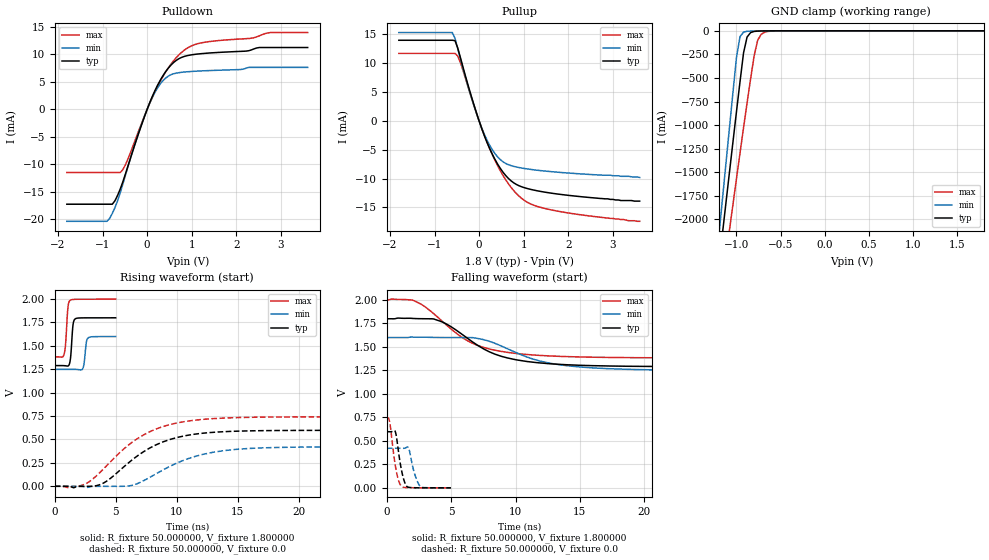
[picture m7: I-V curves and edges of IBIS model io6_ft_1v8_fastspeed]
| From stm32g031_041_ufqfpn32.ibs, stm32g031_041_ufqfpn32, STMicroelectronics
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|   Model io6_ft_1v8_fastspeed
[Model]  io6_ft_1v8_fastspeed
Model_type I/O
Polarity   Non-Inverting
Enable   Active-Low
Vinl =   0.540000V
Vinh =   1.260000V
Vmeas =  0.900000V
Cref =   30.000000pF
Rref =   100.000000M
Vref =   0.0V
C_comp   1.277600pF   1.236700pF   1.315100pF
[Temperature Range]   25.000000   -40.000000   0.125000k
[Pullup Reference]   1.800000V   1.600000V   2.000000V
[Pulldown Reference]   0.0V   0.0V   0.0V
[POWER Clamp Reference]   1.800000V   1.600000V   2.000000V
[GND Clamp Reference]   0.0V   0.0V   0.0V
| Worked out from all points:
|   slope of the pulldown table from 0 to 0.27 V, typ, clamps not added: 54.7 ohm
|   slope of the pullup table from 0 to 0.27 V, typ, clamps not added: 50.6 ohm
|   GND clamp passes 1 mA (typ) near -0.66 V on its own axis
|   rising waveform, R_fixture 50.000000, V_fixture 1.800000: 20-80 % time 165ps typ, 169ps min, 180ps max; typ from 1.29 V to 1.8 V
|   rising waveform, R_fixture 50.000000, V_fixture 0.0: 20-80 % time 4.07ns typ, 4.38ns min, 4.26ns max; typ from 0 V to 0.598 V
|   falling waveform, R_fixture 50.000000, V_fixture 1.800000: 20-80 % time 3.95ns typ, 4.46ns min, 3.82ns max; typ from 1.8 V to 1.29 V
|   falling waveform, R_fixture 50.000000, V_fixture 0.0: 20-80 % time 437ps typ, 479ps min, 450ps max; typ from 0.598 V to 0 V
[Pulldown]
|Voltage   I(typ)   I(min)   I(max)
-1.8V     -17.22mA   -20.33mA   -11.45mA
-900mV    -17.22mA   -20.33mA   -11.45mA
-720mV    -16.58mA   -17.82mA   -11.45mA
-600mV    -14.41mA   -15.08mA   -11.45mA
-480mV    -11.58mA   -11.79mA   -9.954mA
0V        10fA       11fA       0A
240mV     4.49mA     3.999mA    4.291mA
480mV     7.563mA    6.085mA    7.612mA
780mV     9.487mA    6.76mA     10.43mA
1.14V     10.08mA    6.976mA    11.96mA
2.76V     11.26mA    7.652mA    13.98mA
3.6V      11.26mA    7.652mA    13.98mA
[Pullup]
|Voltage   I(typ)   I(min)   I(max)
-1.8V     14mA       15.34mA    11.72mA
-600mV    14mA       15.34mA    11.72mA
-540mV    13.93mA    14.32mA    11.72mA
-420mV    11.01mA    10.78mA    10.15mA
-180mV    4.421mA    4.232mA    4.225mA
60mV      -1.349mA   -1.244mA   -1.314mA
300mV     -5.831mA   -5.038mA   -5.917mA
600mV     -9.499mA   -7.385mA   -10.25mA
960mV     -11.43mA   -8.172mA   -13.47mA
1.32V     -12.13mA   -8.557mA   -14.86mA
2.16V     -13.03mA   -9.116mA   -16.14mA
3.6V      -13.9mA    -9.8mA     -17.4mA
[GND_clamp]
|Voltage   I(typ)   I(min)   I(max)
-1.8V     -7.471A    -7.973A    -7.298A
-1.2V     -2.489A    -2.18A     -2.954A
-1.16V    -2.16A     -1.797A    -2.674A
-1.08V    -1.505A    -1.034A    -2.118A
-1V       -857.9mA   -283.1mA   -1.568A
-960mV    -540.4mA   -62.14mA   -1.296A
-920mV    -234.4mA   -13.75mA   -1.028A
-880mV    -66.29mA   -4.855mA   -765.3mA
-800mV    -6.505mA   -2.056mA   -266mA
-760mV    -3.074mA   -1.45mA    -100.4mA
-680mV    -1.215mA   -557.1uA   -14.19mA
1.8V      0A         0A         0A
[POWER_clamp]
|Voltage   I(typ)   I(min)   I(max)
-1.8V     0A         0A         0A
0V        0A         0A         0A
[Ramp]
| variable   typ   min   max
dV/dt_r  0.35857/4.06140n   0.25271/4.37750n   0.44174/4.25525n
dV/dt_f  0.30570/3.93750n   0.21030/4.44000n   0.37008/3.81562n
R_load = 50.000000
[Rising Waveform]
R_fixture= 50.000000
V_fixture= 1.800000
V_fixture_min= 1.600000
V_fixture_max= 2.000000
|time   V(typ)   V(min)   V(max)
0s        1.29V      1.249V     1.383V
770.8ps   1.288V     1.249V     1.413V
880.9ps   1.287V     1.249V     1.515V
1.081ns   1.285V     1.249V     1.912V
1.241ns   1.328V     1.249V     1.985V
1.491ns   1.721V     1.249V     1.996V
1.662ns   1.787V     1.249V     1.997V
2.302ns   1.799V     1.26V      1.998V
2.713ns   1.8V       1.583V     1.999V
4.985ns   1.8V       1.6V       2V
[Rising Waveform]
R_fixture= 50.000000
V_fixture= 0.0
V_fixture_min= 0.0
V_fixture_max= 0.0
|time   V(typ)   V(min)   V(max)
0s        -1.302uV   812.8nV    119.3nV
2.222ns   -952uV     -326.2uV   10.6mV
3.664ns   15.81mV    -606.4uV   142.4mV
5.586ns   199.7mV    -268.5uV   391mV
6.847ns   332.1mV    33.02mV    515.7mV
8.348ns   445.7mV    137.2mV    614.2mV
10.21ns   527.2mV    259.8mV    681.7mV
12.97ns   576.4mV    363.7mV    722.9mV
15.86ns   591.8mV    403.6mV    736.3mV
29.91ns   597.8mV    421.2mV    742.3mV
[Falling Waveform]
R_fixture= 50.000000
V_fixture= 1.800000
V_fixture_min= 1.600000
V_fixture_max= 2.000000
|time   V(typ)   V(min)   V(max)
0s        1.8V       1.6V       2V
2.042ns   1.803V     1.605V     1.996V
3.664ns   1.797V     1.601V     1.852V
4.805ns   1.731V     1.6V       1.713V
6.306ns   1.588V     1.6V       1.563V
7.928ns   1.451V     1.561V     1.48V
9.369ns   1.383V     1.481V     1.442V
11.89ns   1.33V      1.35V      1.41V
14.95ns   1.305V     1.287V     1.394V
29.91ns   1.29V      1.249V     1.383V
[Falling Waveform]
R_fixture= 50.000000
V_fixture= 0.0
V_fixture_min= 0.0
V_fixture_max= 0.0
|time   V(typ)   V(min)   V(max)
0s        597.8mV    421.2mV    742.3mV
230.2ps   597.3mV    421.3mV    694.6mV
660.7ps   598mV      421.5mV    238.2mV
870.9ps   424.3mV    421.4mV    97.81mV
1.101ns   217.7mV    421mV      23.34mV
1.381ns   61.79mV    422.4mV    4.382mV
1.682ns   6.505mV    426.3mV    2.064mV
2.172ns   1.368mV    144.8mV    1.225mV
2.623ns   599.4uV    13.21mV    861.6uV
4.985ns   -1.302uV   812.8nV    119.3nV
